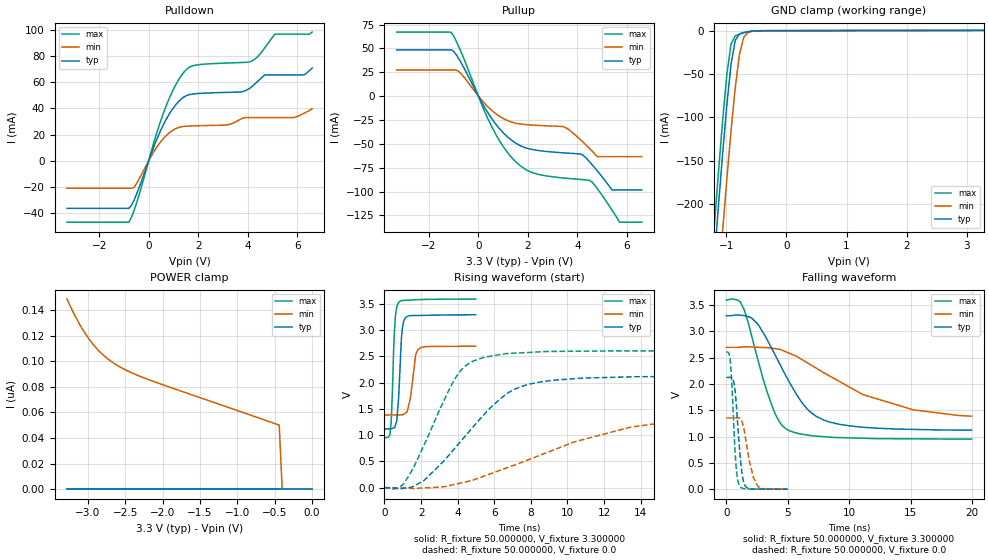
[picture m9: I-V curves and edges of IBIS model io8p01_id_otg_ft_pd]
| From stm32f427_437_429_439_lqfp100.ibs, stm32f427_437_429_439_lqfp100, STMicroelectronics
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|   Model io8p01_id_otg_ft_pd
[Model]  io8p01_id_otg_ft_pd
Model_type I/O
Polarity   Non-Inverting
Enable   Active-Low
Vinl =   0.990000V
Vinh =   2.310000V
Vmeas =  1.650000V
Cref =   50.000000pF
Rref =   100.000000M
Vref =   0.0V
C_comp   2.283100pF   2.214500pF   2.357400pF
[Temperature Range]   25.000000   0.125000k   -40.000000
[Pullup Reference]   3.300000V   2.700000V   3.600000V
[Pulldown Reference]   0.0V   0.0V   0.0V
[POWER Clamp Reference]   3.300000V   2.700000V   3.600000V
[GND Clamp Reference]   0.0V   0.0V   0.0V
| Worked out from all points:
|   slope of the pulldown table from 0 to 0.495 V, typ, clamps not added: 20.9 ohm
|   slope of the pullup table from 0 to 0.495 V, typ, clamps not added: 22.6 ohm
|   GND clamp passes 1 mA (typ) near -0.62 V on its own axis
|   rising waveform, R_fixture 50.000000, V_fixture 3.300000: 20-80 % time 192ps typ, 292ps min, 166ps max; typ from 1.12 V to 3.29 V
|   rising waveform, R_fixture 50.000000, V_fixture 0.0: 20-80 % time 3.35ns typ, 6.84ns min, 2.1ns max; typ from 0 V to 2.12 V
|   falling waveform, R_fixture 50.000000, V_fixture 3.300000: 20-80 % time 3.18ns typ, 6.86ns min, 2ns max; typ from 3.29 V to 1.12 V
|   falling waveform, R_fixture 50.000000, V_fixture 0.0: 20-80 % time 432ps typ, 670ps min, 341ps max; typ from 2.12 V to 0 V
[Pulldown]
|Voltage   I(typ)   I(min)   I(max)
-3.3V     -36.46mA   -21.1mA    -47.09mA
-800mV    -36.46mA   -21.1mA    -47.09mA
-600mV    -30.5mA    -20.54mA   -38.68mA
700mV     31.39mA    19.11mA    41.7mA
1.2V      45.14mA    25.37mA    61.74mA
1.6V      50.34mA    26.49mA    71.04mA
3.1V      52.26mA    27.25mA    74.74mA
4.1V      55.69mA    32.98mA    75.78mA
4.7V      65.7mA     32.98mA    86.67mA
5.1V      65.7mA     32.98mA    96.88mA
6.3V      65.85mA    36.49mA    96.88mA
6.6V      70.9mA     39.7mA     98.46mA
[Pullup]
|Voltage   I(typ)   I(min)   I(max)
-3.3V     48.54mA    27.43mA    67.16mA
-1.1V     48.54mA    27.43mA    66.89mA
-700mV    35.13mA    23.47mA    46.35mA
500mV     -22.06mA   -14mA      -30.03mA
1.5V      -49.1mA    -28.3mA    -68.56mA
2.2V      -56.04mA   -30.32mA   -80.35mA
3.5V      -59.53mA   -32.65mA   -85.92mA
4.5V      -69.07mA   -55.13mA   -88.38mA
4.8V      -78.23mA   -63.4mA    -96.83mA
5.4V      -98.3mA    -63.4mA    -119.6mA
5.7V      -98.3mA    -63.4mA    -132.1mA
6.6V      -98.3mA    -63.4mA    -132.1mA
[GND_clamp]
|Voltage   I(typ)   I(min)   I(max)
-3.3V     -2.316A    -2.396A    -2.289A
-1.2V     -265.5mA   -356.1mA   -227.2mA
-1.13V    -202.7mA   -292.9mA   -164.2mA
-1.06V    -142.2mA   -231.2mA   -104.1mA
-990mV    -86mA      -171.6mA   -50.76mA
-920mV    -38.84mA   -115.5mA   -15.35mA
-850mV    -11.15mA   -65.63mA   -6.09mA
-780mV    -3.853mA   -27.45mA   -3.961mA
-710mV    -2.153mA   -7.739mA   -2.46mA
-640mV    -1.209mA   -2.169mA   -1.292mA
-570mV    -580.3uA   -846.3uA   -542.8uA
3.28V     342.5uA    239.2uA    398.5uA
[POWER_clamp]
|Voltage   I(typ)   I(min)   I(max)
-3.28V    0A         148.5nA    0A
-3.2V     0A         138.6nA    0A
-3.12V    0A         129.7nA    0A
-3.04V    0A         122nA      0A
-2.96V    0A         115.3nA    0A
-2.8V     0A         105.1nA    0A
-2.6V     0A         96.44nA    0A
-2.4V     0A         90.52nA    0A
-2.16V    0A         84.97nA    0A
-440mV    0A         50.04nA    0A
-400mV    0A         0A         0A
0V        0A         0A         0A
[Ramp]
| variable   typ   min   max
dV/dt_r  1.27680/3.35260n   0.79668/6.84360n   1.56396/2.09438n
dV/dt_f  1.30116/3.18503n   0.74142/6.82211n   1.58591/1.99712n
R_load = 50.000000
[Rising Waveform]
R_fixture= 50.000000
V_fixture= 3.300000
V_fixture_min= 2.700000
V_fixture_max= 3.600000
|time   V(typ)   V(min)   V(max)
0s        1.121V     1.387V     952.6mV
300.3ps   1.123V     1.387V     1.013V
370.4ps   1.125V     1.387V     1.277V
500.5ps   1.139V     1.387V     2.629V
590.6ps   1.179V     1.387V     3.237V
760.8ps   1.661V     1.385V     3.521V
940.9ps   2.91V      1.389V     3.563V
1.161ns   3.244V     1.425V     3.57V
1.842ns   3.281V     2.639V     3.583V
4.985ns   3.295V     2.695V     3.594V
[Rising Waveform]
R_fixture= 50.000000
V_fixture= 0.0
V_fixture_min= 0.0
V_fixture_max= 0.0
|time   V(typ)   V(min)   V(max)
0s        358.5uV    205.7uV    685uV
1.081ns   -9.495mV   -1.989mV   89.14mV
2.162ns   137.9mV    -2.087mV   812.3mV
3.724ns   702.4mV    54.6mV     1.997V
4.244ns   914.3mV    95.69mV    2.261V
4.885ns   1.174V     150.4mV    2.418V
6.687ns   1.794V     379mV      2.556V
8.408ns   2.008V     605.8mV    2.587V
13.41ns   2.111V     1.151V     2.607V
19.94ns   2.124V     1.354V     2.607V
[Falling Waveform]
R_fixture= 50.000000
V_fixture= 3.300000
V_fixture_min= 2.700000
V_fixture_max= 3.600000
|time   V(typ)   V(min)   V(max)
0s        3.295V     2.695V     3.594V
880.9ps   3.309V     2.695V     3.598V
1.441ns   3.297V     2.705V     3.409V
2.563ns   3.133V     2.696V     2.457V
3.684ns   2.673V     2.679V     1.6V
4.965ns   2.098V     2.597V     1.131V
6.567ns   1.524V     2.403V     1.029V
8.368ns   1.277V     2.154V     989.6mV
15.22ns   1.136V     1.507V     956.3mV
19.94ns   1.121V     1.387V     952.6mV
[Falling Waveform]
R_fixture= 50.000000
V_fixture= 0.0
V_fixture_min= 0.0
V_fixture_max= 0.0
|time   V(typ)   V(min)   V(max)
0s        2.124V     1.354V     2.607V
300.3ps   2.125V     1.354V     2.467V
450.5ps   2.114V     1.354V     1.946V
620.6ps   2.01V      1.354V     1.075V
840.8ps   1.482V     1.356V     291.2mV
1.041ns   825.1mV    1.349V     76.62mV
1.451ns   98.44mV    1.113V     9.651mV
1.852ns   11.84mV    543.1mV    3.861mV
2.573ns   2.018mV    46.86mV    1.869mV
4.985ns   358.5uV    205.7uV    685uV
